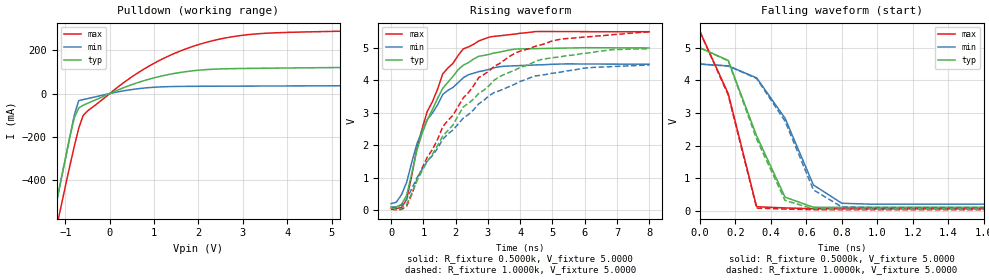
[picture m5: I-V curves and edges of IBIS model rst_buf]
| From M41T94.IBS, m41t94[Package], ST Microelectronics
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|   Model rst_buf
[Model]   rst_buf
Model_type   Open_drain
Polarity   Inverting
Vmeas =   1.5000V
Cref =1.000e-10F
Rref =   0.6450k
Vref =   1.7300V
C_comp   4.5900pF   4.4300pF   4.7800pF
[Temperature Range]   27.0000   85.0000   -40.0000
[Voltage Range]   4.0000V   2.7000V   5.5000V
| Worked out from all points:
|   slope of the pulldown table from 0 to 0.6 V, typ, clamps not added: 12.4 ohm
|   rising waveform, R_fixture 0.5000k, V_fixture 5.0000: 20-80 % time 1.2ns typ, 1.16ns min, 1.14ns max; typ from 0.108 V to 5 V
|   rising waveform, R_fixture 1.0000k, V_fixture 5.0000: 20-80 % time 2.31ns typ, 2.36ns min, 2.28ns max; typ from 0.054 V to 4.98 V
|   falling waveform, R_fixture 0.5000k, V_fixture 5.0000: 20-80 % time 222ps typ, 242ps min, 181ps max; typ from 5 V to 0.107 V
|   falling waveform, R_fixture 1.0000k, V_fixture 5.0000: 20-80 % time 219ps typ, 241ps min, 182ps max; typ from 5 V to 0.054 V
[Pulldown]
| voltage   I(typ)   I(min)   I(max)
-4V       -3.3A      -3.3A      -3.38A
-1.3V     -600mA     -600mA     -714mA
-1V       -300mA     -300mA     -426.8mA
-800mV    -112.2mA   -100mA     -243.5mA
-700mV    -66.89mA   -32.57mA   -160.4mA
-600mV    -53.66mA   -27.79mA   -101.3mA
-500mV    -45.06mA   -23.29mA   -79.97mA
500mV     41.34mA    18.54mA    77.23mA
1.3V      86.65mA    31.87mA    170.6mA
2.2V      110.7mA    33.62mA    237.4mA
3.5V      116.9mA    34.7mA     277.8mA
8V        131.5mA    41.4mA     305.1mA
[Ramp]
| variable   typ   min   max
dV/dt_r   2.3613/1.5550n   1.5645/1.7774n   3.2711/1.4687n
dV/dt_f   2.3604/0.1421n   1.5649/0.1952n   3.2698/0.1009n
R_load = 0.6450k
[Rising Waveform]
R_fixture = 0.5000k
V_fixture = 5.0000
V_fixture_min = 4.5000
V_fixture_max = 5.5000
| time   V(typ)   V(min)   V(max)
0s        107.5mV    204.8mV    64.64mV
160ps     106.5mV    248.4mV    56.62mV
480ps     457.7mV    854.9mV    325.1mV
800ps     1.852V     2.048V     1.916V
1.12ns    2.782V     2.798V     3.046V
1.6ns     3.758V     3.566V     4.199V
2.24ns    4.468V     4.085V     4.972V
3.04ns    4.803V     4.341V     5.332V
3.84ns    4.963V     4.449V     5.428V
8ns       4.999V     4.498V     5.5V
[Rising Waveform]
R_fixture = 1.0000k
V_fixture = 5.0000
V_fixture_min = 4.5000
V_fixture_max = 5.5000
| time   V(typ)   V(min)   V(max)
0s        53.63mV    100.7mV    32.31mV
480ps     181.5mV    340.8mV    124mV
800ps     908.1mV    999.8mV    940.4mV
1.6ns     2.284V     2.185V     2.572V
2.24ns    3.186V     2.841V     3.466V
2.72ns    3.601V     3.281V     4.091V
3.2ns     4.012V     3.631V     4.435V
4ns       4.398V     3.969V     4.905V
5.12ns    4.711V     4.234V     5.242V
8ns       4.976V     4.473V     5.496V
[Falling Waveform]
R_fixture = 0.5000k
V_fixture = 5.0000
V_fixture_min = 4.5000
V_fixture_max = 5.5000
| time   V(typ)   V(min)   V(max)
0s        5V         4.5V       5.5V
160ps     4.612V     4.445V     3.591V
320ps     2.298V     4.078V     124.8mV
480ps     418.4mV    2.84V      88.5mV
640ps     108.7mV    792.8mV    65.38mV
800ps     107.5mV    230.7mV    64.94mV
960ps     107.4mV    204.3mV    64.53mV
8ns       107.4mV    204.6mV    64.9mV
[Falling Waveform]
R_fixture = 1.0000k
V_fixture = 5.0000
V_fixture_min = 4.5000
V_fixture_max = 5.5000
| time   V(typ)   V(min)   V(max)
0s        5V         4.5V       5.5V
160ps     4.6V       4.442V     3.547V
320ps     2.2V       4.059V     81.74mV
480ps     319.5mV    2.751V     53.54mV
640ps     58.57mV    641.9mV    33.09mV
800ps     53.49mV    117.5mV    32.59mV
960ps     54.22mV    100.7mV    32.24mV
8ns       53.97mV    100.7mV    32.55mV
